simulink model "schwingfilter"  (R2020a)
settings: Solver=ode45  StartTime=0.0  StopTime=100  RelTol=1e-3  EnableMultiTasking=on
libraries: simulink_extras x1

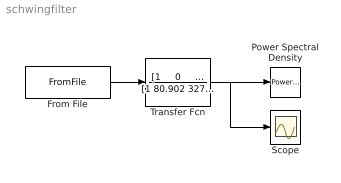
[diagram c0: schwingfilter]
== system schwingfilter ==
  From File : FromFile  FileName=schwingung.mat  SampleTime=0
  Power Spectral Density : simulink_extras/Additional Sinks/Power Spectral Density  npts=1024  fftpts=1024  HowOften=64  sampleT=0.05
  Scope : Scope
  Transfer Fcn : TransferFcn  Numerator="[1     0     0     0     0     0]"  Denominator=[1 80.902 3272.5 81814 1.2641e6 9.7656e6]
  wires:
  From File/1 -> Transfer Fcn/1
  Transfer Fcn/1 -> Power Spectral Density/1, Scope/1
